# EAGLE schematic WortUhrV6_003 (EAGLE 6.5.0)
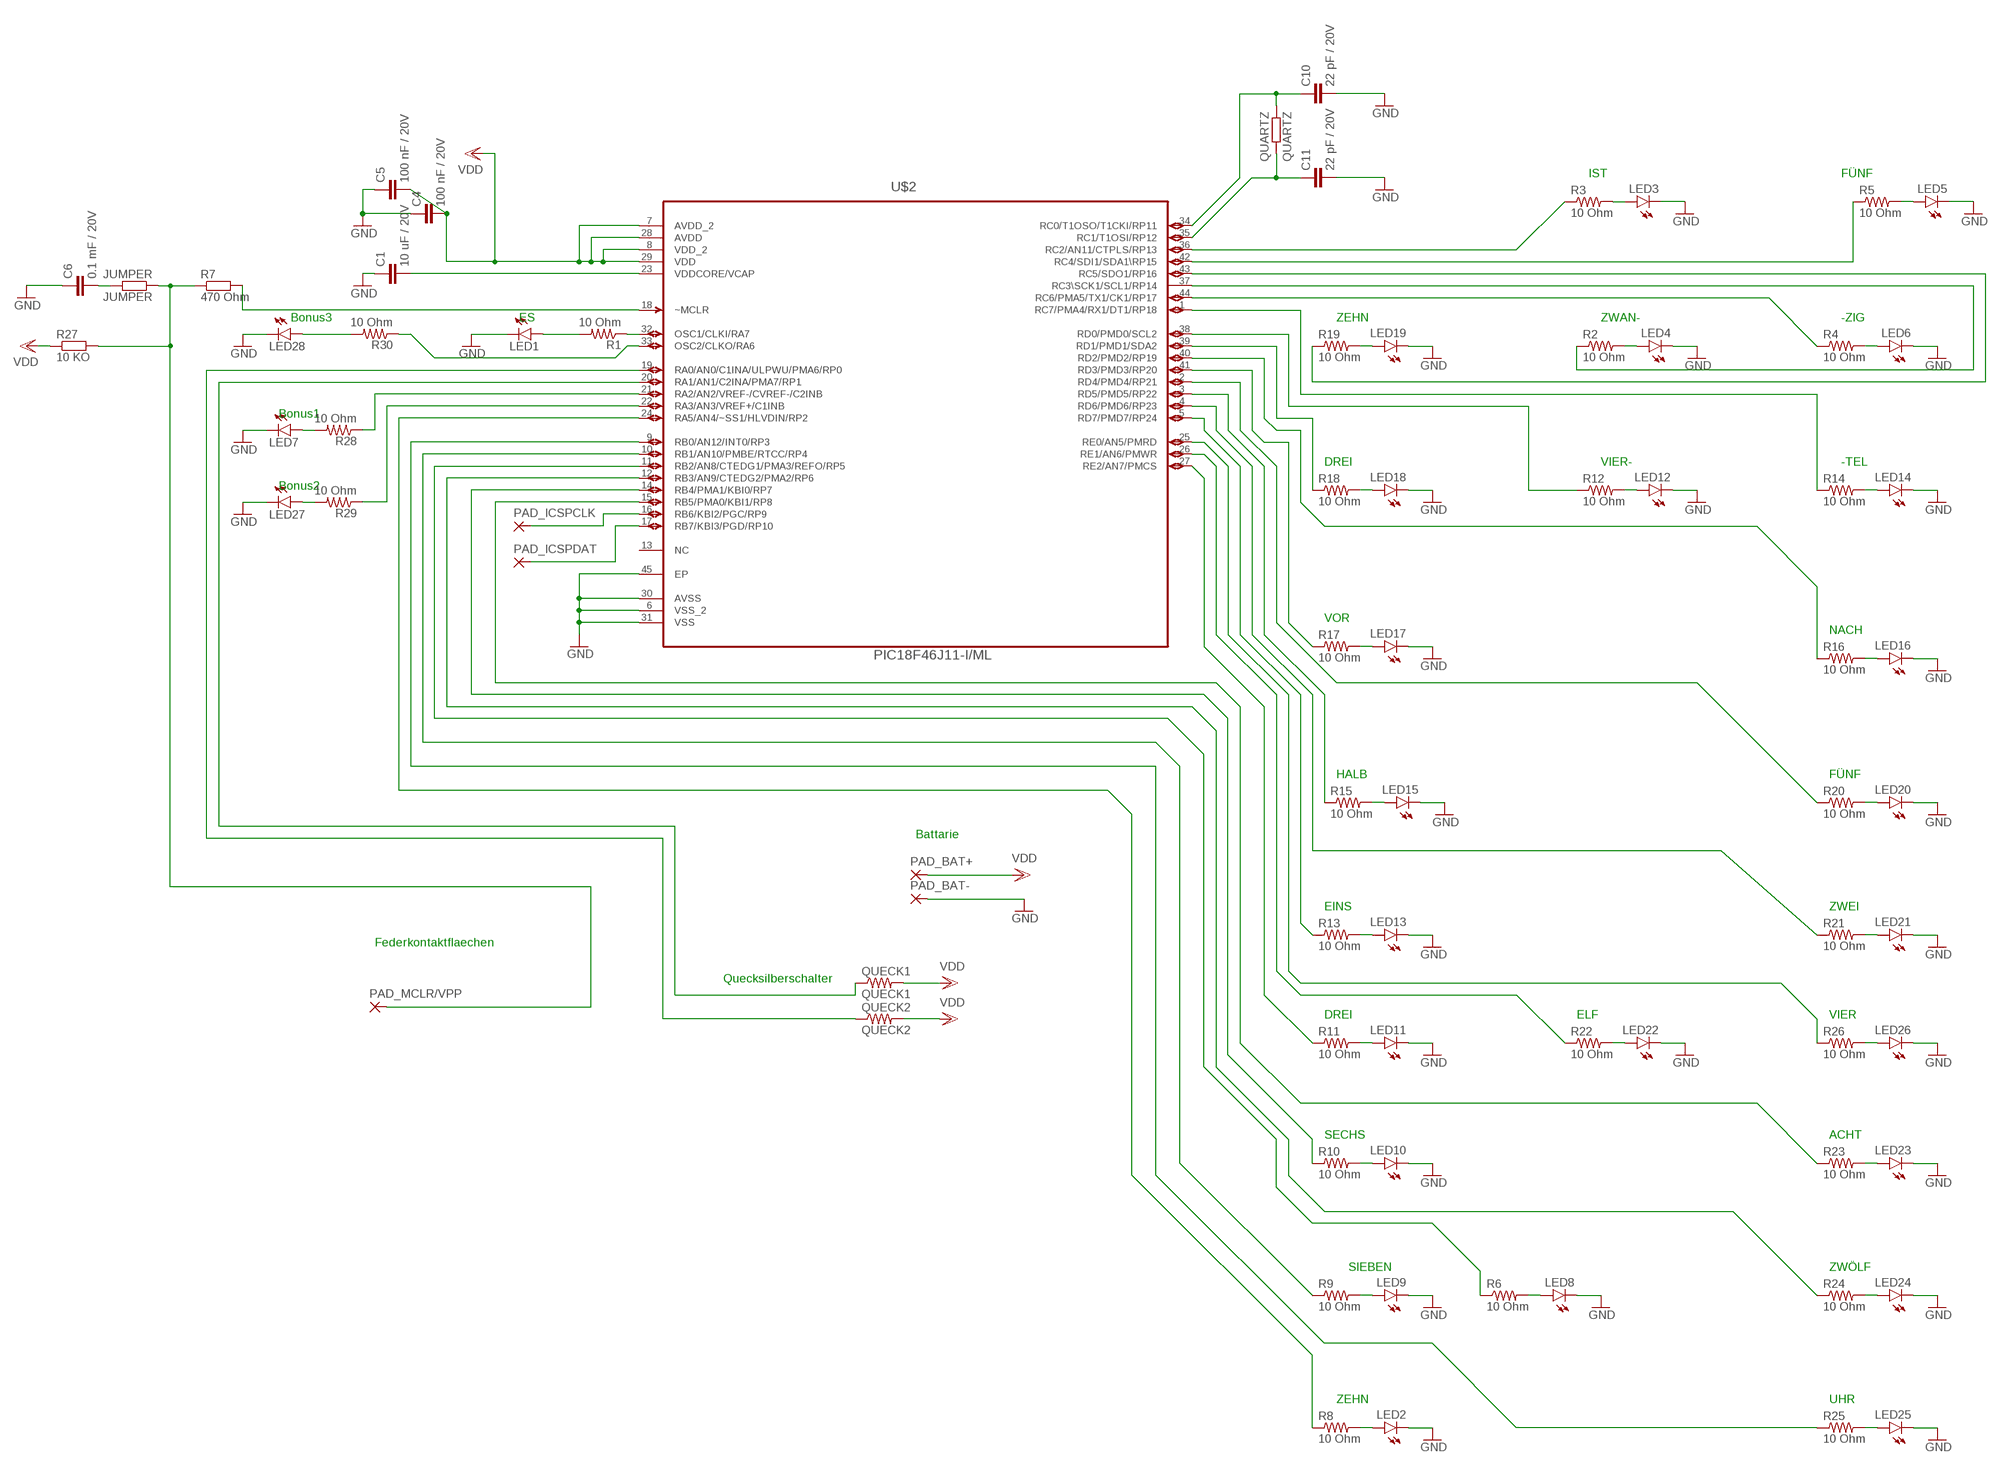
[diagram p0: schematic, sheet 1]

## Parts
C1  10 uF / 20V  C-EUC0603  [C0603]
C4  100 nF / 20V  C-EUC0603  [C0603]
C5  100 nF / 20V  C-EUC0603  [C0603]
C6  0.1 mF / 20V  C-EUC0603  [C0603]
C10  22 pF / 20V  C-EUC0603  [C0603]
C11  22 pF / 20V  C-EUC0603  [C0603]
JUMPER  JUMPER  R-EU_R0603  [R0603]
LED1  LED0603  [LED-0603]
LED2  LED0603  [LED-0603]
LED3  LED0603  [LED-0603]
LED4  LED0603  [LED-0603]
LED5  LED0603  [LED-0603]
LED6  LED0603  [LED-0603]
LED7  LED0603  [LED-0603]
LED8  LED0603  [LED-0603]
LED9  LED0603  [LED-0603]
LED10  LED0603  [LED-0603]
LED11  LED0603  [LED-0603]
LED12  LED0603  [LED-0603]
LED13  LED0603  [LED-0603]
LED14  LED0603  [LED-0603]
LED15  LED0603  [LED-0603]
LED16  LED0603  [LED-0603]
LED17  LED0603  [LED-0603]
LED18  LED0603  [LED-0603]
LED19  LED0603  [LED-0603]
LED20  LED0603  [LED-0603]
LED21  LED0603  [LED-0603]
LED22  LED0603  [LED-0603]
LED23  LED0603  [LED-0603]
LED24  LED0603  [LED-0603]
LED25  LED0603  [LED-0603]
LED26  LED0603  [LED-0603]
LED27  LED0603  [LED-0603]
LED28  LED0603  [LED-0603]
PAD_BAT+  SMD2  [SMD1,27-2,54]
PAD_BAT-  SMD2  [SMD1,27-2,54]
PAD_ICSPCLK  SMD2  [SMD1,27-2,54]
PAD_ICSPDAT  SMD2  [SMD1,27-2,54]
PAD_MCLR/VPP  SMD2  [SMD1,27-2,54]
QUARTZ  QUARTZ  R-EU_R0603  [R0603]
QUECK1  QUECK1  RESISTOR0603  [0603-RES]
QUECK2  QUECK2  RESISTOR0603  [0603-RES]
R1  10 Ohm  RESISTOR0603  [0603-RES]
R2  10 Ohm  RESISTOR0603  [0603-RES]
R3  10 Ohm  RESISTOR0603  [0603-RES]
R4  10 Ohm  RESISTOR0603  [0603-RES]
R5  10 Ohm  RESISTOR0603  [0603-RES]
R6  10 Ohm  RESISTOR0603  [0603-RES]
R7  470 Ohm  R-EU_R0603  [R0603]
R8  10 Ohm  RESISTOR0603  [0603-RES]
R9  10 Ohm  RESISTOR0603  [0603-RES]
R10  10 Ohm  RESISTOR0603  [0603-RES]
R11  10 Ohm  RESISTOR0603  [0603-RES]
R12  10 Ohm  RESISTOR0603  [0603-RES]
R13  10 Ohm  RESISTOR0603  [0603-RES]
R14  10 Ohm  RESISTOR0603  [0603-RES]
R15  10 Ohm  RESISTOR0603  [0603-RES]
R16  10 Ohm  RESISTOR0603  [0603-RES]
R17  10 Ohm  RESISTOR0603  [0603-RES]
R18  10 Ohm  RESISTOR0603  [0603-RES]
R19  10 Ohm  RESISTOR0603  [0603-RES]
R20  10 Ohm  RESISTOR0603  [0603-RES]
R21  10 Ohm  RESISTOR0603  [0603-RES]
R22  10 Ohm  RESISTOR0603  [0603-RES]
R23  10 Ohm  RESISTOR0603  [0603-RES]
R24  10 Ohm  RESISTOR0603  [0603-RES]
R25  10 Ohm  RESISTOR0603  [0603-RES]
R26  10 Ohm  RESISTOR0603  [0603-RES]
R27  10 KO  R-EU_R0603  [R0603]
R28  10 Ohm  RESISTOR0603  [0603-RES]
R29  10 Ohm  RESISTOR0603  [0603-RES]
R30  10 Ohm  RESISTOR0603  [0603-RES]
U$2  PIC18F46J11-I/ML  [QFN65P800X800X100-45N]

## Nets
GND: C1.1 C4.1 C5.1 C6.1 C10.2 C11.2 LED1.C LED2.C LED3.C LED4.C LED5.C LED6.C LED7.C LED8.C LED9.C LED10.C LED11.C LED12.C LED13.C LED14.C LED15.C LED16.C LED17.C LED18.C LED19.C LED20.C LED21.C LED22.C LED23.C LED24.C LED25.C LED26.C LED27.C LED28.C PAD_BAT-.1(P) U$2.6(VSS_2) U$2.30(AVSS) U$2.31(VSS) U$2.45(EP)
N$1: LED16.A R16.2
N$2: LED8.A R6.2
N$3: LED2.A R8.2
N$4: LED20.A R20.2
N$5: LED9.A R9.2
N$6: LED10.A R10.2
N$7: LED11.A R11.2
N$8: LED13.A R13.2
N$9: LED15.A R15.2
N$10: LED17.A R17.2
N$11: LED18.A R18.2
N$12: LED19.A R19.2
N$13: LED4.A R2.2
N$14: LED21.A R21.2
N$15: LED6.A R4.2
N$16: LED12.A R12.2
N$17: LED14.A R14.2
N$18: LED22.A R22.2
N$19: LED23.A R23.2
N$20: LED24.A R24.2
N$21: LED25.A R25.2
N$22: LED26.A R26.2
N$23: R1.1 U$2.32(OSC1/CLKI/RA7)
N$24: R3.1 U$2.36(RC2/AN11/CTPLS/RP13)
N$25: LED7.A R28.2
N$26: R19.1 U$2.43(RC5/SDO1/RP16)
N$27: R2.1 U$2.37(RC3\SCK1/SCL1/RP14)
N$28: LED1.A R1.2
N$29: LED3.A R3.2
N$30: R4.1 U$2.44(RC6/PMA5/TX1/CK1/RP17)
N$31: R14.1 U$2.1(RC7/PMA4/RX1/DT1/RP18)
N$32: R12.1 U$2.38(RD0/PMD0/SCL2)
N$33: R18.1 U$2.39(RD1/PMD1/SDA2)
N$34: R16.1 U$2.40(RD2/PMD2/RP19)
N$35: R17.1 U$2.41(RD3/PMD3/RP20)
N$36: R20.1 U$2.2(RD4/PMD4/RP21)
N$37: LED27.A R29.2
N$38: R15.1 U$2.3(RD5/PMD5/RP22)
N$39: R21.1 U$2.4(RD6/PMD6/RP23)
N$40: R13.1 U$2.5(RD7/PMD7/RP24)
N$41: R26.1 U$2.25(RE0/AN5/PMRD)
N$42: R22.1 U$2.26(RE1/AN6/PMWR)
N$43: R11.1 U$2.27(RE2/AN7/PMCS)
N$44: R23.1 U$2.15(RB5/PMA0/KBI1/RP8)
N$45: R10.1 U$2.14(RB4/PMA1/KBI0/RP7)
N$46: R24.1 U$2.12(RB3/AN9/CTEDG2/PMA2/RP6)
N$47: R6.1 U$2.11(RB2/AN8/CTEDG1/PMA3/REFO/RP5)
N$48: R9.1 U$2.10(RB1/AN10/PMBE/RTCC/RP4)
N$49: JUMPER.1 PAD_MCLR/VPP.1(P) R7.1 R27.2
N$50: R25.1 U$2.9(RB0/AN12/INT0/RP3)
N$51: PAD_ICSPCLK.1(P) U$2.16(RB6/KBI2/PGC/RP9)
N$52: R8.1 U$2.24(RA5/AN4/~SS1/HLVDIN/RP2)
N$53: PAD_ICSPDAT.1(P) U$2.17(RB7/KBI3/PGD/RP10)
N$54: QUECK1.1 U$2.20(RA1/AN1/C2INA/PMA7/RP1)
N$55: LED5.A R5.2
N$56: QUECK2.1 U$2.19(RA0/AN0/C1INA/ULPWU/PMA6/RP0)
N$57: R5.1 U$2.42(RC4/SDI1/SDA1\RP15)
N$58: R29.1 U$2.22(RA3/AN3/VREF+/C1INB)
N$59: R28.1 U$2.21(RA2/AN2/VREF-/CVREF-/C2INB)
N$60: C1.2 U$2.23(VDDCORE/VCAP)
N$61: R7.2 U$2.18(~MCLR)
N$62: C6.2 JUMPER.2
N$64: LED28.A R30.2
N$65: R30.1 U$2.33(OSC2/CLKO/RA6)
N$68: C11.1 QUARTZ.2 U$2.35(RC1/T1OSI/RP12)
N$69: C10.1 QUARTZ.1 U$2.34(RC0/T1OSO/T1CKI/RP11)
VDD: C4.2 C5.2 PAD_BAT+.1(P) QUECK1.2 QUECK2.2 R27.1 U$2.7(AVDD_2) U$2.8(VDD_2) U$2.28(AVDD) U$2.29(VDD)
Unconnected: U$2.13(NC)

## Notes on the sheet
- IST | FÜNF
- Bonus3 | ES | ZEHN | ZWAN- | -ZIG
- Bonus1
- DREI | VIER- | -TEL
- Bonus2
- VOR
- NACH
- HALB | FÜNF
- Battarie
- EINS | ZWEI
- Federkontaktflaechen
- Quecksilberschalter
- DREI | ELF | VIER
- SECHS | ACHT
- SIEBEN | ZWÖLF
- ZEHN | UHR

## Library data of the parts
C1 C4-C6 C10 C11 = rcl:C-EU: CAPACITOR, European symbol
JUMPER QUARTZ R7 R27 = rcl:R-EU_: RESISTOR, European symbol
LED1-LED28 = SparkFun-LED:LED: LEDs
PAD_BAT+ PAD_BAT- PAD_ICSPCLK PAD_ICSPDAT PAD_MCLR/VPP = wirepad:SMD2: SMD PAD
QUECK1 QUECK2 R1-R6 R8-R26 R28-R30 = SparkFun-Resistors:RESISTOR: Resistor
U$2 = Microchip_PIC18F46J11:PIC18F46J11-I/ML: 8BIT MCU; DESCRIPTION: 8BIT MCU; MPN: PIC18F46J11-I/Ml; OC_FARNELL: 1698920; OC_NEWARK: 98M1829; PACKAGE: QFN-44; SUPPLIER: Microchip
